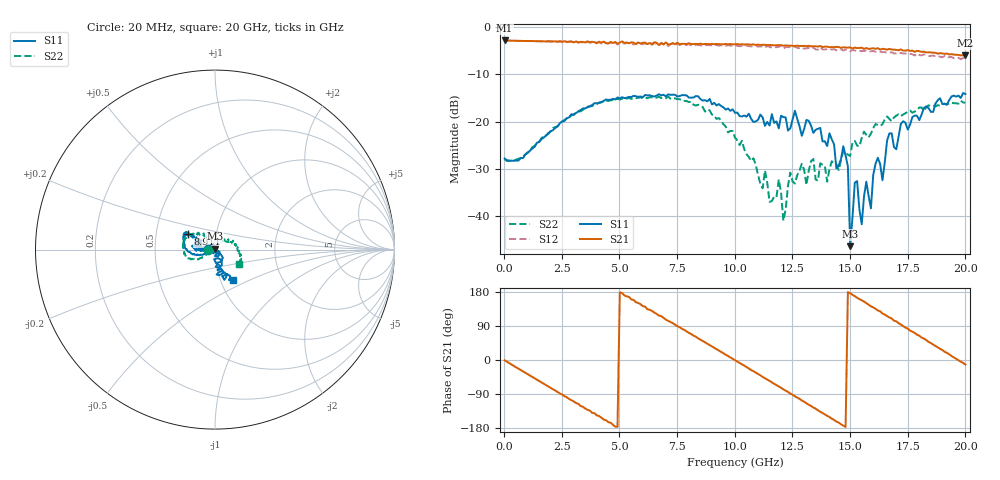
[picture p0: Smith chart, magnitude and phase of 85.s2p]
!Agilent Technologies,N5230A,US43500223,A.07.50.48
!Agilent N5230A: A.07.50.48
!Date: Tuesday, November 17, 2015 12:45:18
!Correction: S11(Full 2 Port(1,2))
!S21(Full 2 Port(1,2))
!S12(Full 2 Port(1,2))
!S22(Full 2 Port(1,2))
!S2P File: Measurements: S11, S21, S12, S22:
# Hz S  dB  R 50
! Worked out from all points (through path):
!   201 points, 20 MHz to 20 GHz, reference 50 ohm
!   highest |S21| = -2.86 dB at 20 MHz (marker M1); lowest = -6.0 dB at 20 GHz (marker M2)
!   group delay of S21, straight-line fit = 101 ps
!   lowest |S11| = -46.3 dB at 15.01 GHz (marker M3), VSWR 1.01, Z = 49.9 + j0.474 ohm
!   |S11| at or under -10 dB: start of sweep to end of sweep
!   |S22| runs from -40.9 to -14.7 dB; largest |S21 - S12| = 0.076
!   S11 on the Smith chart (normalised r, x): 20 MHz: 0.92, +0.00; 8.911 GHz: 0.73, +0.13; 20 GHz: 1.15, -0.40
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2e7  -27.81 178.9  -2.86 -0.7  -2.86 -0.8  -27.96 -179.9
1.9181e9  -22.40 -157.7  -3.01 -69.9  -3.04 -71.0  -22.58 -149.1
3.4166e9  -17.22 -172.2  -3.18 -123.4  -3.43 -124.9  -17.50 -156.4
5.1149e9  -14.85 166.3  -3.07 176.6  -3.23 173.7  -15.17 -174.2
6.7133e9  -14.22 154.8  -3.83 117.1  -3.94 115.1  -14.75 165.7
8.9111e9  -15.22 150.3  -3.65 39.5  -3.84 35.8  -17.63 134.2
1.001e10  -18.15 151.1  -3.67 -0.4  -3.88 -3.7  -23.38 118.9
1.15085e10  -20.83 158.9  -3.81 -55.1  -4.20 -58.5  -36.94 133.3
1.19081e10  -21.42 171.4  -3.84 -70.1  -4.19 -73.9  -32.25 160.5
1.21079e10  -19.04 162.4  -3.95 -77.4  -4.55 -82.0  -40.93 160.5
1.24076e10  -21.42 176.2  -3.93 -88.5  -4.28 -93.3  -30.76 -178.8
1.34066e10  -22.37 175.5  -4.10 -125.3  -4.38 -128.7  -27.90 166.8
1.4006e10  -25.16 -173.1  -4.16 -147.1  -4.69 -150.3  -32.70 142.6
1.47053e10  -25.20 -166.9  -4.32 -173.2  -4.99 -176.9  -26.18 92.2
1.49051e10  -29.47 147.0  -4.37 179.2  -4.86 175.1  -27.00 77.4
1.5005e10  -46.31 100.7  -4.30 176.0  -5.16 172.1  -27.26 62.6
1.52048e10  -32.89 -110.9  -4.37 168.5  -4.97 164.0  -24.08 64.0
1.55045e10  -41.69 53.9  -4.39 157.7  -5.11 153.2  -23.48 46.6
1.57043e10  -32.69 -60.8  -4.45 150.0  -5.01 145.8  -22.80 49.4
1.59041e10  -38.32 -54.3  -4.60 141.6  -5.14 139.2  -22.53 38.6
1.67033e10  -22.50 -66.8  -4.63 112.3  -5.42 108.9  -19.44 24.6
2e10  -14.16 -58.3  -6.03 -12.2  -6.58 -17.5  -16.01 -30.4
